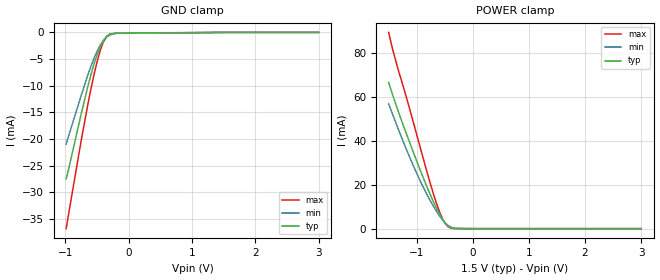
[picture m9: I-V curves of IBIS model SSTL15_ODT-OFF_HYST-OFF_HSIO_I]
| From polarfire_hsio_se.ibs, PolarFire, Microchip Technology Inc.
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|   Model SSTL15_ODT-OFF_HYST-OFF_HSIO_I
[Model]   SSTL15_ODT-OFF_HYST-OFF_HSIO_I
Model_type   Input
Vinl =   0.65
Vinh =   0.85
|   typ   min   max
C_comp_pullup   1.335e-12   1.335e-12   1.380e-12
C_comp_pulldown  1.335e-12   1.335e-12   1.380e-12
[Temperature Range]  25C   100C   -40C
[Voltage Range]  1.5   1.425   1.575
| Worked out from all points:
|   GND clamp passes 1 mA (typ) near -0.36 V on its own axis
|   POWER clamp passes 1 mA (typ) near -0.43 V on its own axis
[GND Clamp]
| Voltage   I(typ)   I(min)   I(max)
-984.4mV  -27.52mA   -20.97mA   -36.83mA
-738.3mV  -14.86mA   -11.51mA   -19.71mA
-639.8mV  -10.04mA   -7.906mA   -13.38mA
-590.6mV  -7.836mA   -6.26mA    -10.46mA
-492.2mV  -4.065mA   -3.445mA   -5.32mA
-443mV    -2.601mA   -2.343mA   -3.27mA
-393.7mV  -1.488mA   -1.478mA   -1.705mA
-344.5mV  -752.5uA   -861uA     -730.3uA
-295.3mV  -360.5uA   -471.5uA   -308.5uA
-196.9mV  -143.7uA   -162.8uA   -160.8uA
-49.22mV  -115.8uA   -98.92uA   -145.6uA
3V        0A         0A         0A
[POWER Clamp]
| Voltage   I(typ)   I(min)   I(max)
-1.5V     66.68mA    56.94mA    89.5mA
-1.427V   60.86mA    52mA       81.61mA
-1.329V   53.48mA    45.42mA    72.38mA
-1.034V   33.05mA    27.15mA    46.05mA
-836.7mV  20.27mA    16.53mA    27.7mA
-689.1mV  11.54mA    9.663mA    14.82mA
-590.6mV  6.461mA    5.759mA    7.506mA
-541.4mV  4.305mA    4.077mA    4.578mA
-443mV    1.22mA     1.505mA    953.6uA
-344.5mV  141uA      346.7uA    82.92uA
-196.9mV  21.95uA    39.89uA    24.88uA
3V        0A         0A         0A
